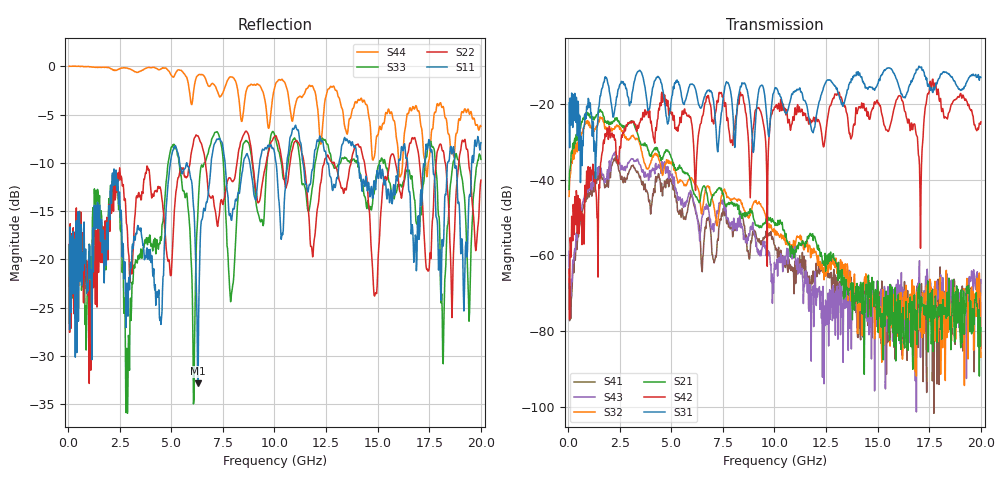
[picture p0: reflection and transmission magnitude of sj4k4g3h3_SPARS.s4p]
! FILE: E:\users\goganessyan\GBX_Backplane\FR408_backplane\1m_INBOUND_FEXT\sj4k4g3h3_SPARS.s4p
# MHZ S RI R 50.00
! FREQ  S11  S12  S13  S14
!  S21  S22  S23  S24
!  S31  S32  S33  S34
!  S41  S42  S43  S44
!  REAL  IMAG  REAL  IMAG  REAL  IMAG  REAL  IMAG
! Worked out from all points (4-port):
!   799 points, 50 MHz to 20 GHz, reference 50 ohm
!   strongest paths, dB at 50 MHz, 5.025 GHz, 10.03 GHz, 15.03 GHz, 20 GHz:
!     S31: -19.8, -18.0, -15.8, -14.5, -13.0
!     S42: -63.7, -23.0, -20.8, -20.0, -24.8
!     S21: -42.6, -34.6, -52.1, -80.3, -79.1
!     S32: -44.5, -35.3, -54.7, -68.3, -86.9
!     S43: -58.9, -39.5, -63.4, -72.5, -66.5
!     S41: -66.3, -41.2, -57.4, -72.1, -80.8
!   lowest |S11| = -32.8 dB at 6.3 GHz (marker M1), VSWR 1.05, Z = 48.4 - j1.59 ohm
!   |S11| at or under -10 dB: start of sweep to 4.96 GHz; 5.751 GHz to 6.93 GHz (1.179 GHz wide, 18.6 % of centre); 14.08 GHz to 16.01 GHz (1.938 GHz wide, 12.9 % of centre)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
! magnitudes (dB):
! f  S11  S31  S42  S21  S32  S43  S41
! 50 MHz  -18.5  -19.8  -63.7  -42.6  -44.5  -58.9  -66.3
! 2.225 GHz  -10.6  -22.8  -28.2  -24.7  -26.8  -33.1  -34.6
! 2.85 GHz  -22.5  -16.6  -26.0  -25.9  -29.5  -36.9  -39.9
! 6.3 GHz  -32.8  -19.7  -29.0  -45.4  -42.4  -51.6  -50.9
! 7.25 GHz  -7.6  -32.7  -19.7  -42.7  -51.5  -48.9  -55.8
! 12.38 GHz  -8.2  -15.7  -31.4  -61.5  -63.4  -78.4  -64.0
! 20 GHz  -7.9  -13.0  -24.8  -79.1  -86.9  -66.5  -80.8
